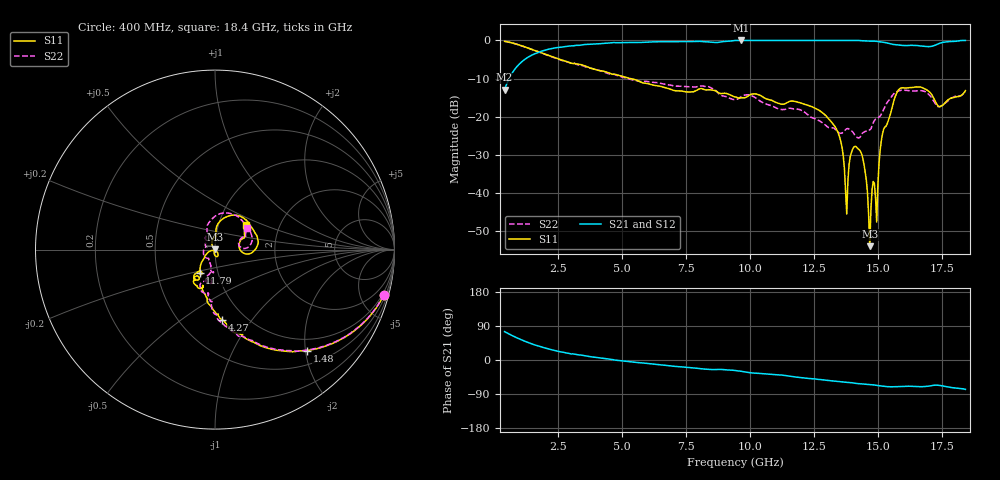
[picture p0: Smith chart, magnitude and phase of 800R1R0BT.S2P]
!  American Technical Ceramics  Date:  6/19/09
!  One Norden Lane
!  Huntington Station,  NY.  11746-2102
!  Tel:  (631) 622-4700  Fax:  (631) 622-4748
!  Part Number  800R1R0BT
!  Description: Ultra-low ESR, NPO  Mounting Orientation: Vertical
!  Application: High RF power Filters, Combiners, Matching networks,
!  Antenna, DC block, Bypass and Couplers
# GHZ S DB R 50
! Freq  |S11|  S11 Ph  |S21|  S21 Ph  |S12|  S12 Ph  |S22|  S22 Ph
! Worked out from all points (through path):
!   401 points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, 400 MHz to 18.4 GHz, reference 50 ohm
!   highest |S21| = -0.01 dB at 9.625 GHz (marker M1); lowest = -12.9 dB at 400 MHz (marker M2)
!   lowest |S11| = -54.0 dB at 14.66 GHz (marker M3), VSWR 1.00, Z = 49.8 + j0.121 ohm
!   |S11| at or under -10 dB: 5.316 GHz to end of sweep
!   |S22| runs from -25.6 to -0.2 dB; largest |S21 - S12| = 0.003
!   S11 on the Smith chart (normalised r, x): 400 MHz: 0.79, -7.47; 1.48 GHz: 0.76, -2.03; 4.27 GHz: 0.79, -0.73; 11.79 GHz: 0.81, -0.22; 18.4 GHz: 1.34, +0.39
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0.4  -0.24 -15.1  -12.92 74.8  -12.93 74.8  -0.24 -15.1
1.48  -2.38 -47.7  -3.80 42.1  -3.80 42.1  -2.40 -47.5
3.415  -6.39 -76.2  -1.18 12.8  -1.18 12.8  -6.57 -77.3
4.27  -8.09 -84.2  -0.78 4.3  -0.78 4.3  -8.25 -87.8
6.43  -11.97 -103.5  -0.34 -12.3  -0.34 -12.3  -11.17 -97.2
9.4  -14.80 -125.3  -0.01 -27.6  -0.01 -27.5  -15.51 -100.4
9.625  -15.07 -122.0  -0.01 -29.6  -0.01 -29.6  -14.80 -95.7
11.785  -16.05 -123.1  -0.01 -45.1  -0.01 -45.1  -17.95 -96.3
12.415  -17.39 -128.2  -0.01 -49.5  -0.01 -49.4  -20.28 -103.2
13.405  -23.87 -148.2  -0.01 -56.4  -0.01 -56.5  -23.96 -123.2
13.765  -45.51 -83.1  -0.01 -58.9  -0.01 -58.9  -23.17 -143.3
13.99  -28.64 -61.9  -0.01 -60.4  -0.01 -60.4  -23.92 -177.4
14.26  -28.73 -83.7  -0.04 -62.5  -0.04 -62.5  -25.54 161.2
14.44  -32.57 -100.6  -0.11 -63.5  -0.10 -63.5  -24.06 145.8
14.665  -53.96 142.7  -0.19 -64.6  -0.18 -64.6  -23.42 132.4
14.98  -38.09 125.6  -0.29 -67.4  -0.28 -67.4  -20.40 116.4
15.16  -24.59 101.0  -0.44 -68.7  -0.43 -68.8  -18.76 113.0
15.43  -20.22 86.8  -0.83 -70.6  -0.81 -70.6  -15.50 96.8
15.88  -12.49 48.1  -1.28 -70.0  -1.27 -70.0  -13.08 60.9
16.78  -12.58 4.4  -1.54 -70.2  -1.53 -70.2  -13.31 16.4
17.41  -17.39 8.3  -0.71 -67.2  -0.70 -67.3  -17.34 15.1
18.4  -13.15 39.3  -0.01 -77.5  -0.01 -77.7  -13.34 33.9
